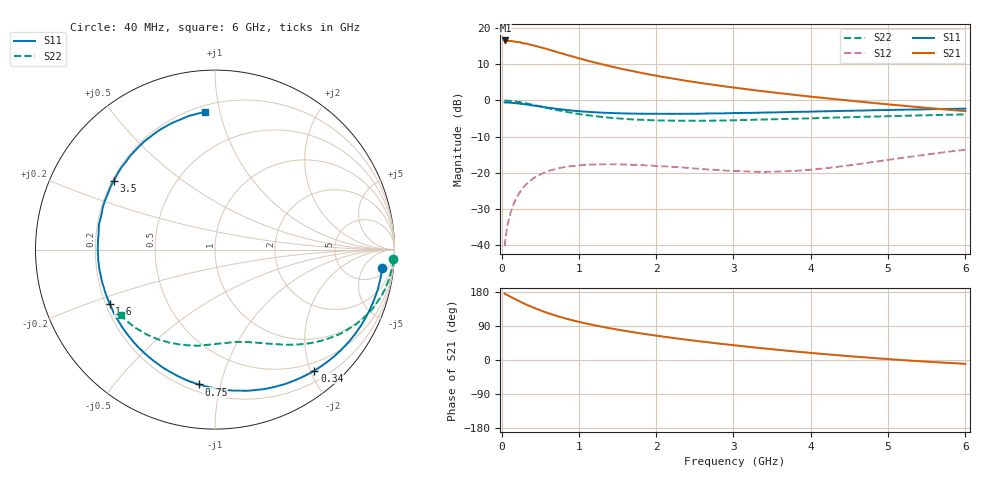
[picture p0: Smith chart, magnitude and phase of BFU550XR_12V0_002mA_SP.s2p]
! Filename:  P:\Prog\Test\Noise\ATS_data\Testdata_Net\03 Spar\BFU550XR_APG2013_45_C05_12p0V_002mA_SP_CM01_D.s2p
! Date/Time: Tue 06/Aug/2013 14:38:18
! BFU550XR_APG2013_45_C05_12p0V_1to35mA_SP_CM01_Bias2_R.s2p
! MDIF S-parameter v. bias file
! BFU550XR_APG2013_45_C05_12p0V_1to35mA_SP_CM01
! Date/time Fri Aug 02 14:58:10 2013
! VAR V_out= 12.0010
! VAR I_out= 2.0000
! VAR V_in= 0.7862
! VAR I_in= 0.0168
! Device data file deembeded for feedlines and parallel
! Original file: \03 Spar\BFU550XR_APG2013_45_C05_12p0V_002mA_SP_CM01_R.s2p
! Feed-files: PR006V01_02082013_Feed1.s2p, PR006V01_02082013_Feed2.s2p
! Parallel-file: PR006V01_02082013_Par.s2p
# MHz S MA R 50
!  Freq-MHz  S11-mag  S11-arg  S21-mag  S21-arg  S12-mag  S12-arg  S22-mag  S22-arg
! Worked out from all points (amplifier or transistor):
!   98 points, 40 MHz to 6 GHz, reference 50 ohm
!   highest |S21| = 16.6 dB at 50 MHz (marker M1)
!   |S21| within 3 dB of that: start of sweep to 687 MHz
!   unconditionally stable (mu >= 1): 3.084 GHz to 4.551 GHz
!   at 300 MHz: K = 0.10, MSG = 19.7 dB, |S12| = -23.7 dB
!   at 1.6 GHz: K = 0.49, MSG = 13.1 dB, |S12| = -17.7 dB
!   at 6 GHz: K = 0.78, MSG = 5.3 dB, |S12| = -13.6 dB
!   S11 on the Smith chart (normalised r, x): 40 MHz: 8, -14; 340 MHz: 0.36, -2.06; 750 MHz: 0.24, -0.86; 1.6 GHz: 0.22, -0.23; 3.5 GHz: 0.21, +0.29; 6 GHz: 0.24, +0.90
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40  0.9383 -6.2  6.725 175.5  0.009681 84.7  0.9956 -3.1
50  0.9369 -7.8  6.735 173.8  0.01204 84.5  0.9946 -4.0
90  0.9334 -13.9  6.61 169.8  0.02166 80.8  0.9879 -7.5
120  0.9282 -18.7  6.639 166.5  0.02864 78.1  0.9829 -10.0
220  0.9071 -33.7  6.404 156.1  0.05038 69.6  0.9504 -17.8
320  0.8782 -47.9  6.106 146.4  0.06917 61.5  0.9088 -25.0
340  0.8728 -50.6  6.028 144.6  0.07247 60.0  0.8995 -26.3
440  0.8414 -63.5  5.661 136.0  0.08741 53.1  0.8538 -32.3
550  0.8079 -76.7  5.263 127.4  0.1001 46.3  0.8021 -38.2
600  0.793 -82.3  5.093 123.8  0.1048 43.6  0.7807 -40.5
750  0.7568 -97.0  4.539 114.2  0.1161 36.6  0.7242 -46.5
900  0.726 -110.1  4.098 105.7  0.1235 30.7  0.6769 -51.5
1050  0.7037 -121.2  3.694 98.3  0.1274 25.9  0.636 -56.0
1300  0.6775 -137.2  3.158 87.7  0.1308 19.6  0.5906 -62.1
1600  0.6611 -152.7  2.668 76.8  0.1299 14.2  0.5549 -68.6
2050  0.6533 -171.2  2.146 62.9  0.1234 9.9  0.5281 -77.1
2500  0.6534 173.5  1.789 50.8  0.1148 8.8  0.5243 -85.2
3100  0.6708 156.2  1.461 36.9  0.105 14.1  0.534 -95.6
3500  0.6818 146.0  1.295 28.4  0.1035 20.5  0.548 -102.8
4100  0.7045 132.0  1.099 16.9  0.113 30.9  0.5695 -113.1
5200  0.7447 109.0  0.844 -0.5  0.1619 39.2  0.6124 -131.8
6000  0.7691 94.2  0.7117 -10.1  0.2084 36.8  0.6406 -145.1
